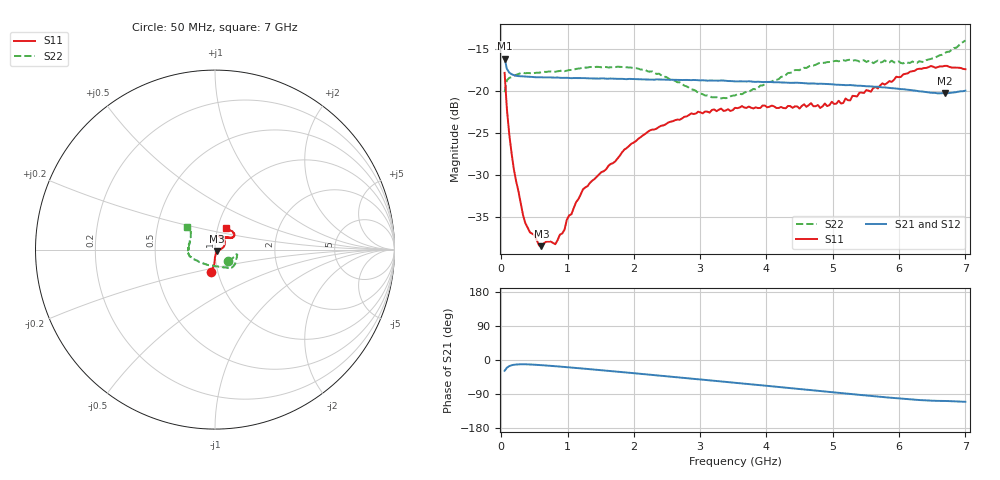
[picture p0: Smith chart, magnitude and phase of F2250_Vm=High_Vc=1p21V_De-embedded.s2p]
! Integrated Device Technology
! Corporate Headquarters
! 6024 Silver Creek Valley Road
! San Jose, CA 95138  USA
! Phone:  1-408-284-8200
! Toll Free:  1-800-223-1366
! Webpage:  http://www.idt.com/
! Timing and RF Division
! 515 Groton Road, Suite 102
! Westford, MA 01886-6024
! Device:  F2250
! Description: Voltage Variable RF Attenuator
! Frequency:  50.0 -  6000.00 MHz
! Package:  3x3 mm Thin QFN Plastic Package: 16 pin
! Ports:  2 RF, 3 DC
!  Pin  1  = GND
!  Pin  2  = NC
!  Pin  3  = RF1  = Port 1
!  Pin  4  = NC
!  Pin  5  = GND
!  Pin  6  = GND
!  Pin  7  = GND
!  Pin  8  = GND
!  Pin  9  = NC
!  Pin 10  = RF2  = Port 2
!  Pin 11  = NC
!  Pin 12  = GND
!  Pin 13  = GND
!  Pin 14  = VCNTRL
!  Pin 15  = VDD
!  Pin 16  = VMODE
! Vcntrl:  1.210 Volts
! Vmode:  +3.300 Volts
! Vdd:  +3.30  Volts
! Current:  1.331 mA
! Data:  The device was measured on a the F2250 evaluation board which has
!  individual transmission lines to the RF pins.  Data was collected
!  using a calibrated network analyzer.  The evaluation board was
!  de-embedded using a TRL calibration technique.
!  The reference plane is the edge of the package pin.
! Misc:  SN 10
!  Action Tracker AT0258
! Date Measured:  2014-11-26
! Date:  2015-10-15  MJV
! Note:
!  Integrated Device Technology supplies this data as a sample of measured
!  data at the package pin for this product.  Your particular data for this
!  product may vary.
!  Data was taken at 25 degrees C.
!  Integrated Device Technology reserves the right to change this data at anytime.
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# GHz S dB R 50
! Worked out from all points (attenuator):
!   201 points, 50 MHz to 7 GHz, reference 50 ohm
!   highest |S21| = -16.18 dB at 50 MHz (marker M1); lowest = -20.3 dB at 6.687 GHz (marker M2)
!   lowest |S11| = -38.5 dB at 606 MHz (marker M3), VSWR 1.02, Z = 50.9 - j0.776 ohm
!   |S11| at or under -10 dB: start of sweep to end of sweep
!   |S22| runs from -20.9 to -14.0 dB; largest |S21 - S12| = 0.00054
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0.05  -17.88 -99.1  -16.18 -28.5  -16.17 -28.4  -20.18 -41.8
0.08475  -22.22 -92.4  -17.42 -20.3  -17.45 -20.3  -18.77 -20.4
0.15425  -27.39 -90.4  -18.04 -13.9  -18.04 -13.9  -18.38 -12.8
0.189  -29.33 -87.5  -18.15 -12.6  -18.16 -12.6  -18.22 -12.4
0.328  -34.81 -70.7  -18.31 -11.3  -18.31 -11.3  -17.89 -12.9
0.43225  -36.86 -66.9  -18.34 -11.8  -18.35 -11.8  -17.92 -14.1
0.606  -38.50 -39.8  -18.41 -13.6  -18.41 -13.6  -17.80 -19.2
0.6755  -37.97 -36.6  -18.42 -14.5  -18.40 -14.5  -17.77 -20.6
0.8145  -38.27 -19.5  -18.45 -16.4  -18.44 -16.4  -17.75 -24.7
0.9535  -36.54 -22.6  -18.48 -18.4  -18.47 -18.4  -17.68 -28.4
0.98825  -35.35 -20.3  -18.47 -18.9  -18.48 -18.9  -17.62 -29.1
1.2315  -31.74 -5.7  -18.51 -22.6  -18.49 -22.6  -17.26 -34.4
1.96125  -26.32 16.6  -18.61 -34.2  -18.62 -34.2  -17.26 -46.5
2.37825  -24.31 27.3  -18.67 -41.0  -18.68 -41.0  -17.98 -54.4
3.07325  -22.48 48.5  -18.78 -52.5  -18.77 -52.6  -20.57 -82.4
3.525  -22.04 61.8  -18.90 -60.1  -18.88 -60.1  -20.57 -113.8
4.7065  -21.85 67.3  -19.14 -80.1  -19.14 -80.1  -17.00 -163.1
5.15825  -21.46 50.6  -19.32 -87.7  -19.32 -87.7  -16.38 -172.1
5.85325  -18.87 35.8  -19.69 -99.3  -19.69 -99.4  -16.64 171.8
6.3745  -17.32 37.8  -20.13 -106.5  -20.15 -106.5  -16.59 154.2
6.68725  -17.05 45.6  -20.33 -108.2  -20.34 -108.3  -15.53 143.7
7  -17.45 62.2  -20.00 -110.3  -20.01 -110.5  -14.03 141.4
